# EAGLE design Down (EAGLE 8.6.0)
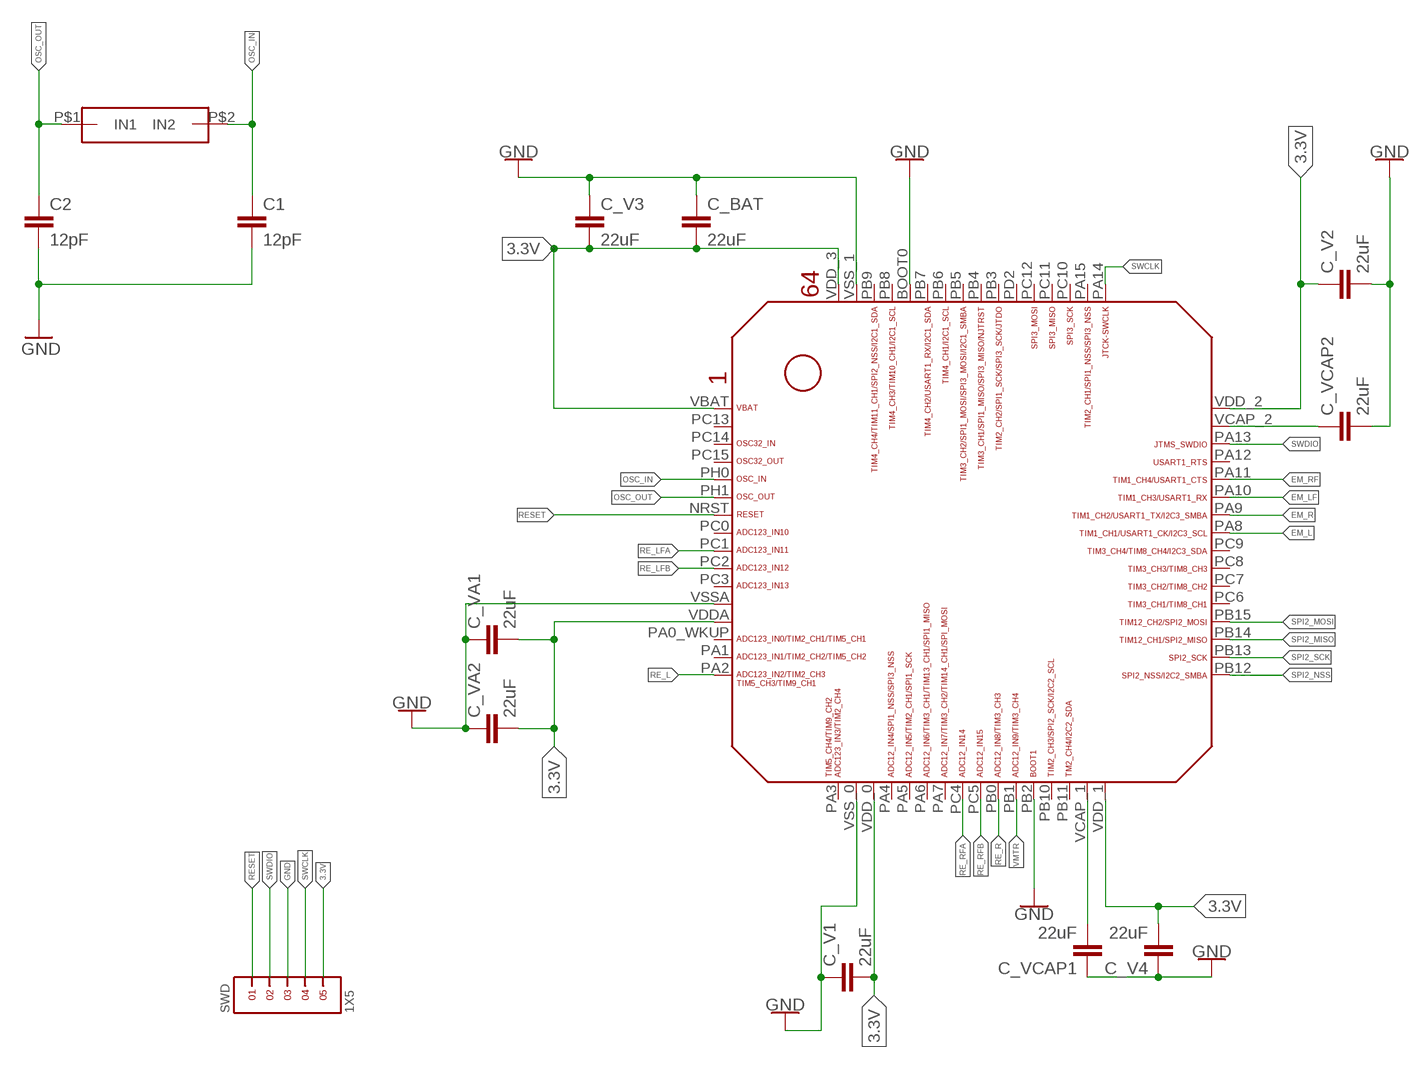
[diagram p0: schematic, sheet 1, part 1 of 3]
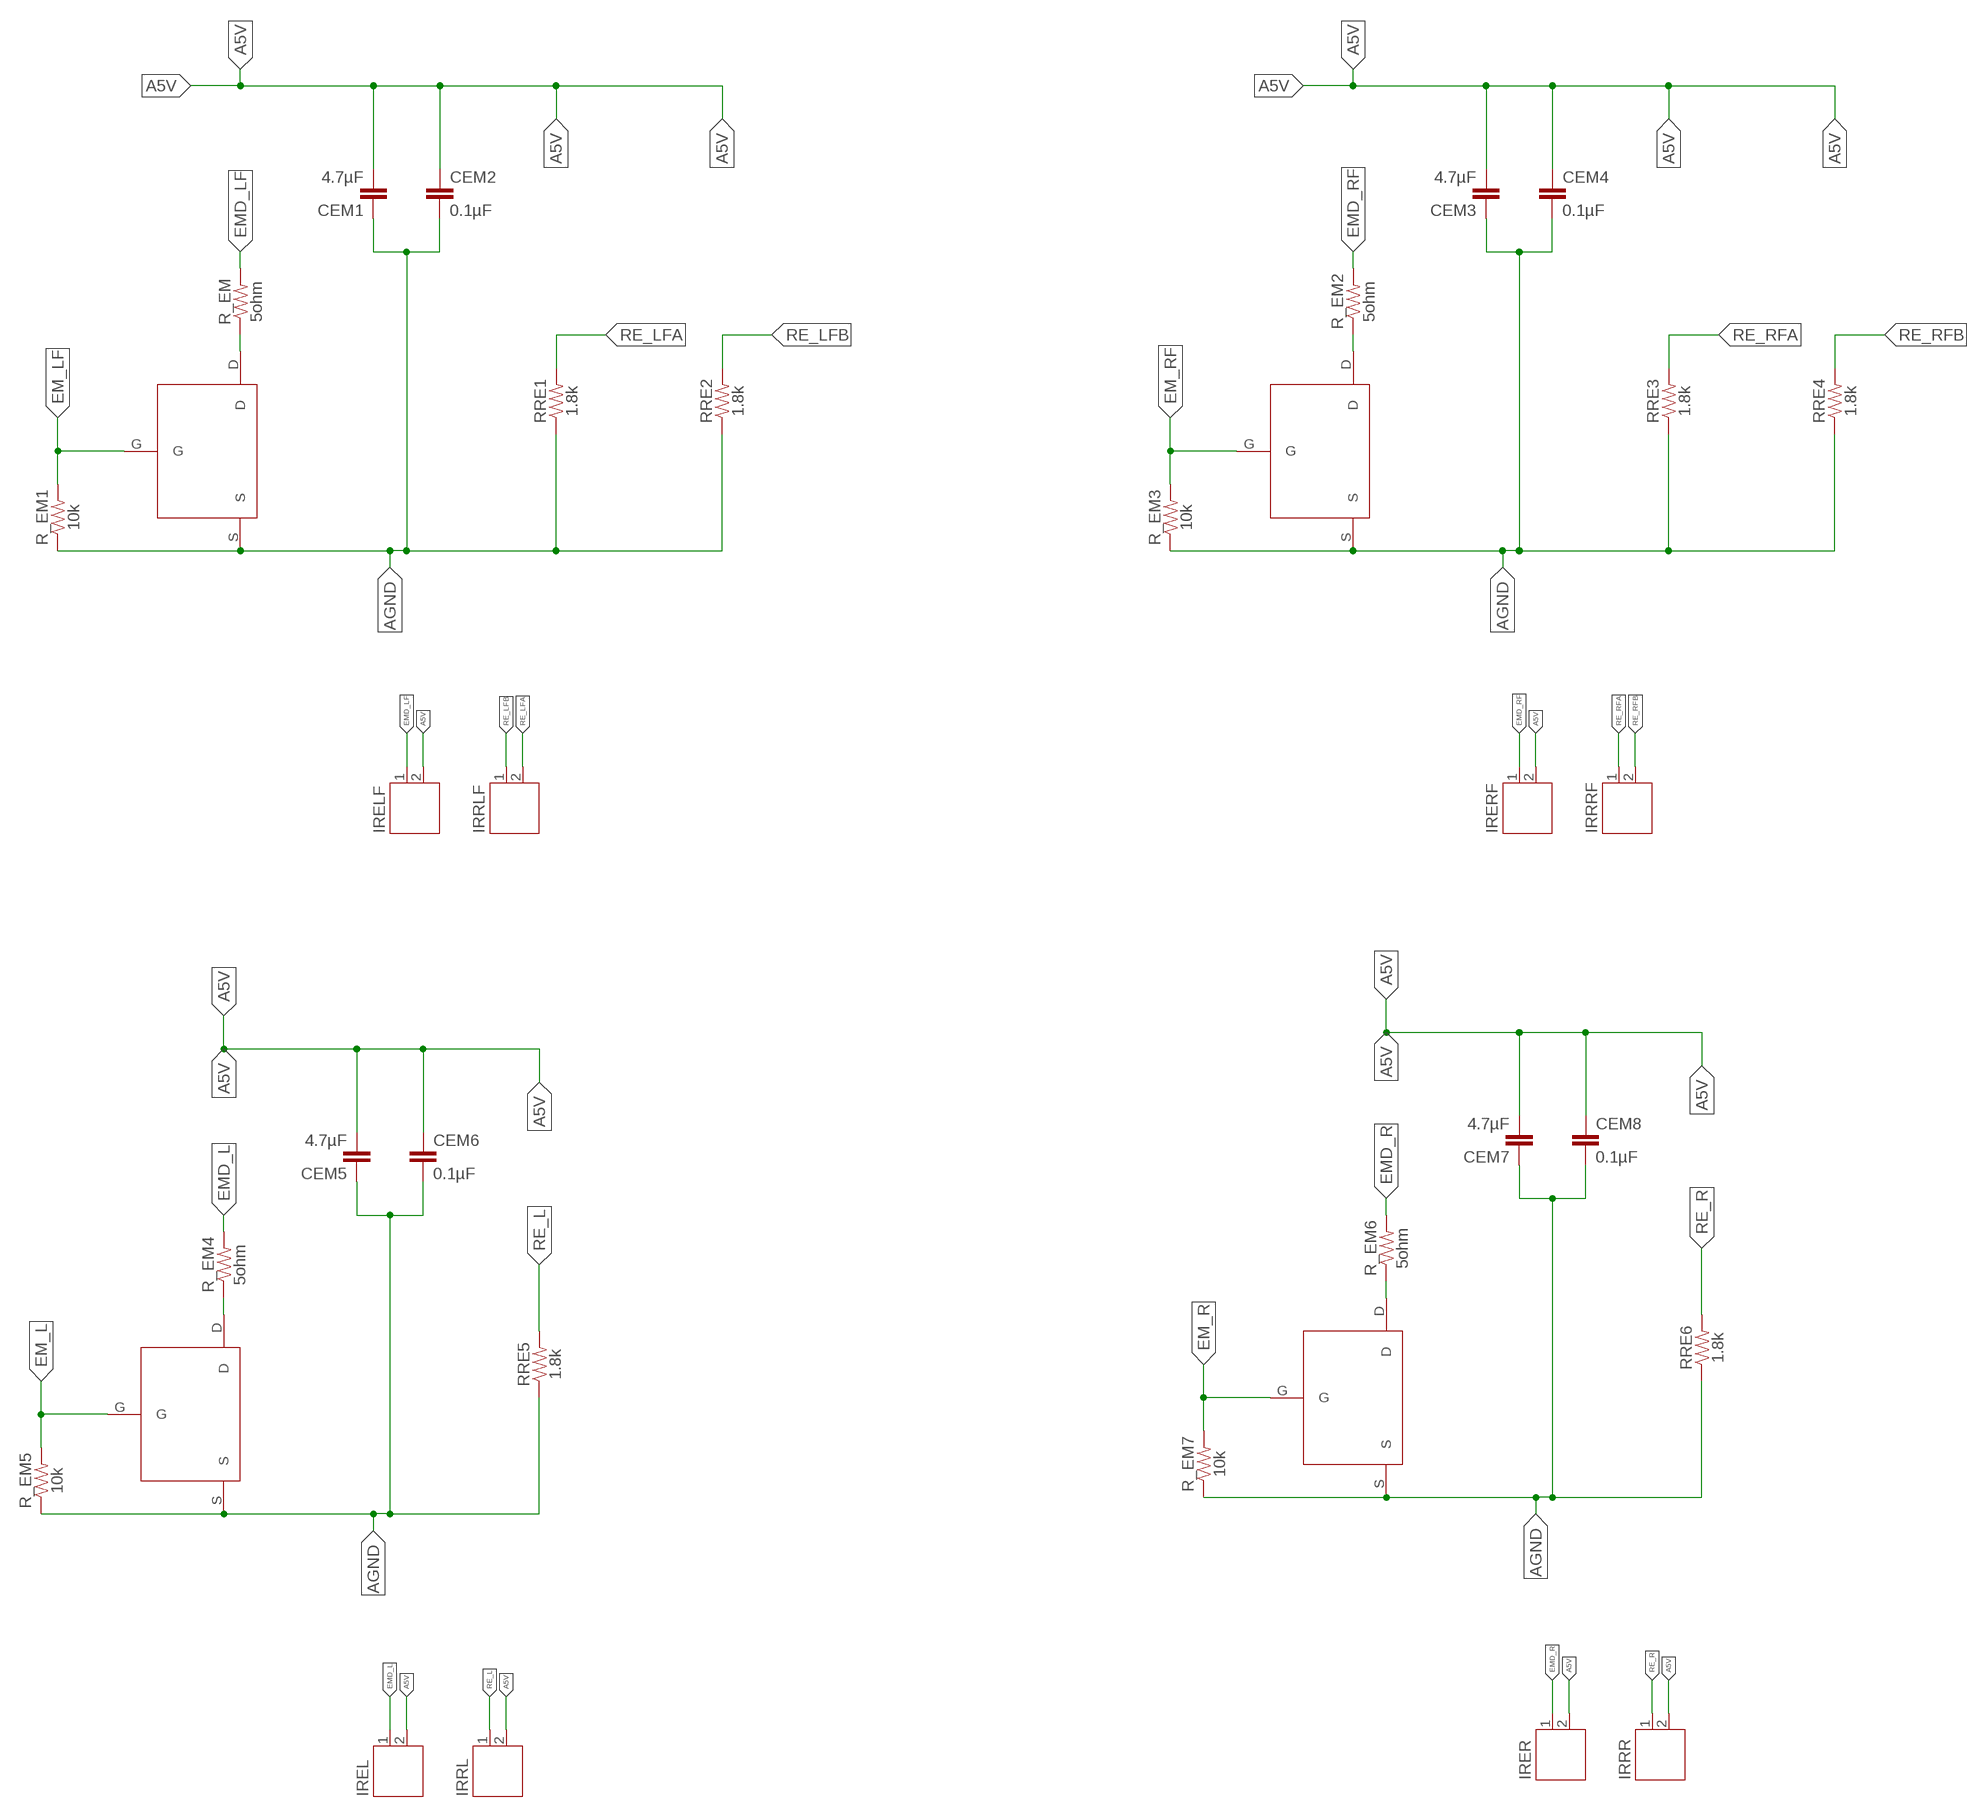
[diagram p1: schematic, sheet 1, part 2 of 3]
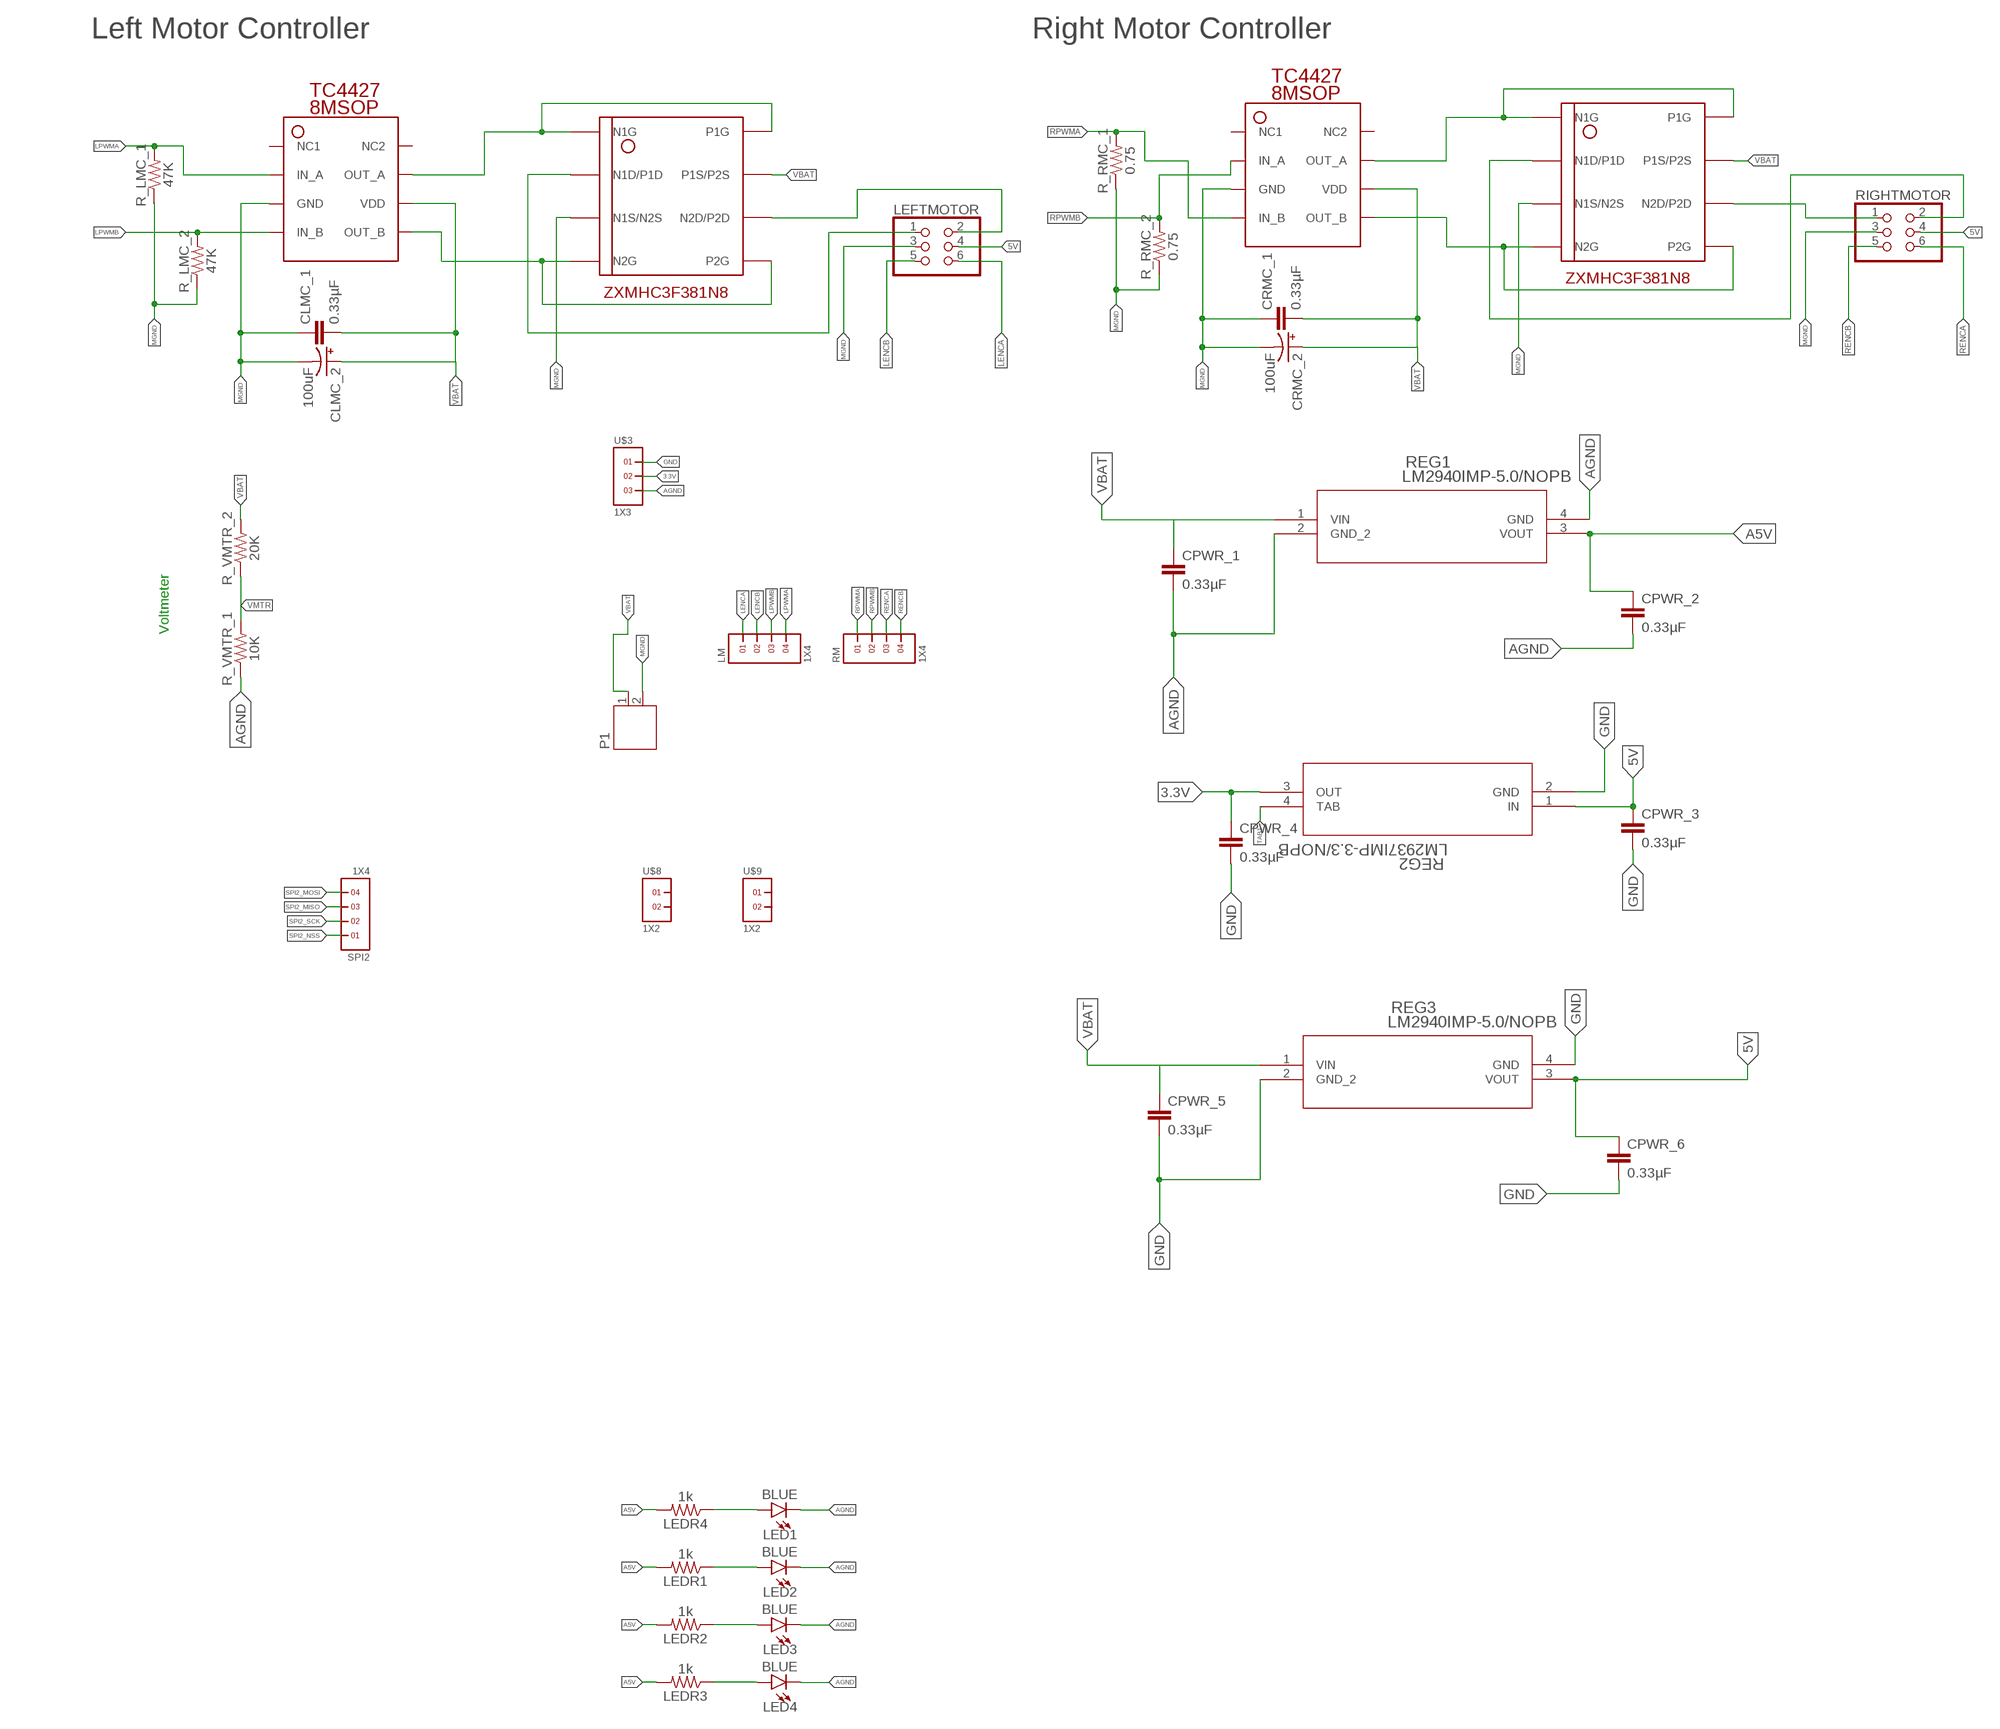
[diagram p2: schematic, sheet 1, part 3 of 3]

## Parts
C1  12pF  22PF-0603-50V-5%  [0603]
C2  12pF  22PF-0603-50V-5%  [0603]
C_BAT  22uF  22UF-0805-6.3V-20%  [0805]
C_V1  22uF  22UF-0805-6.3V-20%  [0805]
C_V2  22uF  22UF-0805-6.3V-20%  [0805]
C_V3  22uF  22UF-0805-6.3V-20%  [0805]
C_V4  22uF  22UF-0805-6.3V-20%  [0805]
C_VA1  22uF  22UF-0805-6.3V-20%  [0805]
C_VA2  22uF  22UF-0805-6.3V-20%  [0805]
C_VCAP1  22uF  22UF-0805-6.3V-20%  [0805]
C_VCAP2  22uF  22UF-0805-6.3V-20%  [0805]
CEM1  4.7µF  0.33UF/330NF-0805-50V-10%  [0805]
CEM2  0.1µF  0.33UF/330NF-0805-50V-10%  [0805]
CEM3  4.7µF  0.33UF/330NF-0805-50V-10%  [0805]
CEM4  0.1µF  0.33UF/330NF-0805-50V-10%  [0805]
CEM5  4.7µF  0.33UF/330NF-0805-50V-10%  [0805]
CEM6  0.1µF  0.33UF/330NF-0805-50V-10%  [0805]
CEM7  4.7µF  0.33UF/330NF-0805-50V-10%  [0805]
CEM8  0.1µF  0.33UF/330NF-0805-50V-10%  [0805]
CLMC_1  0.33µF  0.33UF/330NF-0805-50V-10%  [0805]
CLMC_2  100uF  100UF-POLAR-EIA7343-10V-10%(TANT)  [EIA7343]
CPWR_1  0.33µF  0.33UF/330NF-0805-50V-10%  [0805]
CPWR_2  0.33µF  0.33UF/330NF-0805-50V-10%  [0805]
CPWR_3  0.33µF  0.33UF/330NF-0805-50V-10%  [0805]
CPWR_4  0.33µF  0.33UF/330NF-0805-50V-10%  [0805]
CPWR_5  0.33µF  0.33UF/330NF-0805-50V-10%  [0805]
CPWR_6  0.33µF  0.33UF/330NF-0805-50V-10%  [0805]
CRMC_1  0.33µF  0.33UF/330NF-0805-50V-10%  [0805]
CRMC_2  100uF  100UF-POLAR-EIA7343-10V-10%(TANT)  [EIA7343]
IREL  JST-PH2  [JST-PH2]
IRELF  JST-PH2  [JST-PH2]
IRER  JST-PH2  [JST-PH2]
IRERF  JST-PH2  [JST-PH2]
IRRL  JST-PH2  [JST-PH2]
IRRLF  JST-PH2  [JST-PH2]
IRRR  JST-PH2  [JST-PH2]
IRRRF  JST-PH2  [JST-PH2]
LED1  BLUE  LED-BLUE1206  [LED-1206]
LED2  BLUE  LED-BLUE1206  [LED-1206]
LED3  BLUE  LED-BLUE1206  [LED-1206]
LED4  BLUE  LED-BLUE1206  [LED-1206]
LEDR1  1k  0.75OHM-0805-1/4W-1%  [0805]
LEDR2  1k  0.75OHM-0805-1/4W-1%  [0805]
LEDR3  1k  0.75OHM-0805-1/4W-1%  [0805]
LEDR4  1k  0.75OHM-0805-1/4W-1%  [0805]
LEFTMOTOR  PINHD-2X3  [2X03]
LM  1X4  [1X4]
P1  JST-PH2  [JST-PH2]
R_EM  5ohm  0.75OHM-0805-1/4W-1%  [0805]
R_EM1  10k  0.75OHM-0805-1/4W-1%  [0805]
R_EM2  5ohm  0.75OHM-0805-1/4W-1%  [0805]
R_EM3  10k  0.75OHM-0805-1/4W-1%  [0805]
R_EM4  5ohm  0.75OHM-0805-1/4W-1%  [0805]
R_EM5  10k  0.75OHM-0805-1/4W-1%  [0805]
R_EM6  5ohm  0.75OHM-0805-1/4W-1%  [0805]
R_EM7  10k  0.75OHM-0805-1/4W-1%  [0805]
R_LMC_1  47K  0.75OHM-0805-1/4W-1%  [0805]
R_LMC_2  47K  0.75OHM-0805-1/4W-1%  [0805]
R_RMC_1  0.75  0.75OHM-0805-1/4W-1%  [0805]
R_RMC_2  0.75  0.75OHM-0805-1/4W-1%  [0805]
R_VMTR_1  10K  0.75OHM-0805-1/4W-1%  [0805]
R_VMTR_2  20K  0.75OHM-0805-1/4W-1%  [0805]
REG1  LM2940IMP-5.0/NOPB  [MP04A]
REG2  LM2937IMP-3.3/NOPB  [MP04A]
REG3  LM2940IMP-5.0/NOPB  [MP04A]
RIGHTMOTOR  PINHD-2X3  [2X03]
RM  1X4  [1X4]
RRE1  1.8k  0.75OHM-0805-1/4W-1%  [0805]
RRE2  1.8k  0.75OHM-0805-1/4W-1%  [0805]
RRE3  1.8k  0.75OHM-0805-1/4W-1%  [0805]
RRE4  1.8k  0.75OHM-0805-1/4W-1%  [0805]
RRE5  1.8k  0.75OHM-0805-1/4W-1%  [0805]
RRE6  1.8k  0.75OHM-0805-1/4W-1%  [0805]
SPI2  1X4  [1X4]
SWD  1X5  [1X5]
U$1  STM32F405/415_LQFP64  [STM32F405/415_LQFP64]
U$2  OSC  [OSC]
U$3  1X3  [1X3]
U$4  MCH3474  [MCH3474]
U$5  MCH3474  [MCH3474]
U$6  MCH3474  [MCH3474]
U$7  MCH3474  [MCH3474]
U$8  1X2  [1X2]
U$9  1X2  [1X2]
U$15  TC4427(8MSOP)  [TC4427(8MSOP)]
U$16  ZXMHC3F381N8  [ZXMHC3F381N8]
U$17  TC4427(8MSOP)  [TC4427(8MSOP)]
U$18  ZXMHC3F381N8  [ZXMHC3F381N8]

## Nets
3.3V: C_BAT.2 C_V1.2 C_V2.1 C_V3.2 C_V4.2 C_VA1.2 C_VA2.2 CPWR_4.1 REG2.3(OUT) SWD.5 U$1.VBAT U$1.VDD_0 U$1.VDD_1 U$1.VDD_2 U$1.VDD_3 U$1.VDDA U$3.2
5V: CPWR_3.1 CPWR_6.1 LEFTMOTOR.4 REG2.1(IN) REG3.3(VOUT) RIGHTMOTOR.4
A5V: CEM1.2 CEM2.1 CEM3.2 CEM4.1 CEM5.2 CEM6.1 CEM7.2 CEM8.1 CPWR_2.1 IREL.2 IRELF.2 IRER.2 IRERF.2 IRRL.2 IRRR.2 LEDR1.2 LEDR2.2 LEDR3.2 LEDR4.2 REG1.3(VOUT)
AGND: CEM1.1 CEM2.2 CEM3.1 CEM4.2 CEM5.1 CEM6.2 CEM7.1 CEM8.2 CPWR_1.2 CPWR_2.2 LED1.C LED2.C LED3.C LED4.C R_EM1.1 R_EM3.1 R_EM5.1 R_EM7.1 R_VMTR_1.1 REG1.2(GND_2) REG1.4(GND) RRE1.1 RRE2.1 RRE3.1 RRE4.1 RRE5.1 RRE6.1 U$3.3 U$4.S U$5.S U$6.S U$7.S
EM_L: R_EM5.2 U$1.PA8 U$4.G
EM_LF: R_EM1.2 U$1.PA10 U$5.G
EM_R: R_EM7.2 U$1.PA9 U$7.G
EM_RF: R_EM3.2 U$1.PA11 U$6.G
EMD_L: IREL.1 R_EM4.2
EMD_LF: IRELF.1 R_EM.2
EMD_R: IRER.1 R_EM6.2
EMD_RF: IRERF.1 R_EM2.2
GND: C1.2 C2.2 C_BAT.1 C_V1.1 C_V2.2 C_V3.1 C_V4.1 C_VA1.1 C_VA2.1 C_VCAP1.1 C_VCAP2.2 CPWR_3.2 CPWR_4.2 CPWR_5.2 CPWR_6.2 REG2.2(GND) REG3.2(GND_2) REG3.4(GND) SWD.3 U$1.BOOT0 U$1.PB2 U$1.VSS_0 U$1.VSS_1 U$1.VSSA U$3.1
L: LEFTMOTOR.1 U$16.N1D/P1D
LENCA: LEFTMOTOR.6 LM.1
LENCB: LEFTMOTOR.5 LM.2
LPWMA: LM.4 R_LMC_1.2 U$15.IN_A
LPWMB: LM.3 R_LMC_2.2 U$15.IN_B
MGND: CLMC_1.1 CLMC_2.C(-) CRMC_1.1 CRMC_2.C(-) LEFTMOTOR.3 P1.2 R_LMC_1.1 R_LMC_2.1 R_RMC_1.1 R_RMC_2.1 RIGHTMOTOR.3 U$15.GND U$16.N1S/N2S U$17.GND U$18.N1S/N2S
N$1: R_EM.1 U$5.D
N$2: R_EM2.1 U$6.D
N$3: R_EM4.1 U$4.D
N$4: R_EM6.1 U$7.D
N$5: LED2.A LEDR1.1
N$6: LED3.A LEDR2.1
N$7: LED4.A LEDR3.1
N$8: LED1.A LEDR4.1
N$28: LEFTMOTOR.2 U$16.N2D/P2D
N$36: RIGHTMOTOR.1 U$18.N2D/P2D
OSC_IN: C1.1 U$1.PH0 U$2.P$2(IN2)
OSC_OUT: C2.1 U$1.PH1 U$2.P$1(IN1)
OUT_A: U$15.OUT_A U$16.N1G U$16.P1G
OUT_B: U$15.OUT_B U$16.N2G U$16.P2G
OUTA: U$17.OUT_A U$18.N1G U$18.P1G
OUTB: U$17.OUT_B U$18.N2G U$18.P2G
R: RIGHTMOTOR.2 U$18.N1D/P1D
RE_L: IRRL.1 RRE5.2 U$1.PA2
RE_LFA: IRRLF.2 RRE1.2 U$1.PC1
RE_LFB: IRRLF.1 RRE2.2 U$1.PC2
RE_R: IRRR.1 RRE6.2 U$1.PB0
RE_RFA: IRRRF.1 RRE3.2 U$1.PC4
RE_RFB: IRRRF.2 RRE4.2 U$1.PC5
RENCA: RIGHTMOTOR.6 RM.3
RENCB: RIGHTMOTOR.5 RM.4
RESET: SWD.1 U$1.NRST
RPWMA: R_RMC_1.2 RM.1 U$17.IN_B
RPWMB: R_RMC_2.2 RM.2 U$17.IN_A
SPI2_MISO: SPI2.3 U$1.PB14
SPI2_MOSI: SPI2.4 U$1.PB15
SPI2_NSS: SPI2.1 U$1.PB12
SPI2_SCK: SPI2.2 U$1.PB13
SWCLK: SWD.4 U$1.PA14
SWDIO: SWD.2 U$1.PA13
TAB1: REG2.4(TAB)
VBAT: CLMC_1.2 CLMC_2.A(+) CPWR_1.1 CPWR_5.1 CRMC_1.2 CRMC_2.A(+) P1.1 R_VMTR_2.2 REG1.1(VIN) REG3.1(VIN) U$15.VDD U$16.P1S/P2S U$17.VDD U$18.P1S/P2S
VCAP_1: C_VCAP1.2 U$1.VCAP_1
VCAP_2: C_VCAP2.1 U$1.VCAP_2
VMTR: R_VMTR_1.2 R_VMTR_2.1 U$1.PB1
Unconnected: U$1.PA0_WKUP(PA0_AKUP) U$1.PA1 U$1.PA3 U$1.PA4 U$1.PA5 U$1.PA6 U$1.PA7 U$1.PA12 U$1.PA15 U$1.PB3 U$1.PB4 U$1.PB5 U$1.PB6 U$1.PB7 U$1.PB8 U$1.PB9 U$1.PB10 U$1.PB11 U$1.PC0 U$1.PC3 U$1.PC6 U$1.PC7 U$1.PC8 U$1.PC9 U$1.PC10 U$1.PC11 U$1.PC12 U$1.PC13 U$1.PC14 U$1.PC15 U$1.PD2 U$8.1 U$8.2 U$9.1 U$9.2 U$15.NC1 U$15.NC2 U$17.NC1 U$17.NC2

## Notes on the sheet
- Left Motor Controller | Right Motor Controller
- Voltmeter

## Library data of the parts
C1 C2 = SparkFun-Capacitors:22PF: 22pF ceramic capacitors; PROD_ID: CAP-07876; VALUE: 22pF
C_BAT C_V1-C_V4 C_VA1 C_VA2 C_VCAP1 C_VCAP2 = SparkFun-Capacitors:22UF: 22µF ceramic capacitors; PROD_ID: CAP-08402
CEM1-CEM8 = SparkFun-Capacitors:0.33UF/330NF: 0.33µF/330nF ceramic capacitors; PROD_ID: CAP-08469; VALUE: 0.33µF
CLMC_1 CPWR_1-CPWR_6 CRMC_1 = SparkFun-Capacitors:0.33UF/330NF: 0.33µF/330nF ceramic capacitors; PROD_ID: CAP-08469
CLMC_2 CRMC_2 = SparkFun-Capacitors:100UF-POLAR: 100µF polarized capacitors; PROD_ID: CAP-07890
IREL IRELF IRER IRERF IRRL IRRLF IRRR IRRRF P1 = jst-ph:JST-PH2
LED1-LED4 = SparkFun-LED:LED-BLUE: Blue SMD LED; PROD_ID: DIO-09911
LEDR1-LEDR4 R_EM R_EM1-R_EM7 R_LMC_1 R_LMC_2 R_VMTR_1 R_VMTR_2 RRE1-RRE6 = SparkFun-Resistors:0.75OHM: 0.75Ω resistor; PROD_ID: RES-08474; VALUE: 0.75
LEFTMOTOR RIGHTMOTOR = pinhead:PINHD-2X3: PIN HEADER
LM RM SPI2 = headers(2mm):1X4
R_RMC_1 R_RMC_2 = SparkFun-Resistors:0.75OHM: 0.75Ω resistor; PROD_ID: RES-08474
REG1 REG3 = LM2940IMP-5.0:LM2940IMP-5.0/NOPB; 3D_LIBRARY_NAME: National_LDO; BASE_PN: LM2940; COMP: TypeLDO; COPYRIGHT: Copyright C 2015 Accelerated Designs. All rights reserved; LIBRARY: ReferenceLM2940IMP; MANUFACTURER_PART_NUMBER: LM2940IMP5.0NOPB; PIN: Count4; SYMBOL: NameLM2940IMP50; TYPE: LM2940IMP5.0; VENDOR: National Semiconductor; VERSION: 1
REG2 = LM2937IMP-3.3:LM2937IMP-3.3/NOPB; COPYRIGHT: Copyright C 2015 Accelerated Designs. All rights reserved; MANUFACTURER_PART_NUMBER: lm2937imp3_3nopb; VENDOR: National Semiconductor
SWD = headers(2mm):1X5
U$1 = STM32F405RG:STM32F405/415_LQFP64
U$2 = Cristal Oscillator:OSC
U$3 = headers(2mm):1X3
U$4-U$7 = MCH3474:MCH3474
U$8 U$9 = headers(2mm):1X2
U$15 U$17 = TC4427(8MSOP):TC4427(8MSOP)
U$16 U$18 = ZXMHC3F381N8:ZXMHC3F381N8

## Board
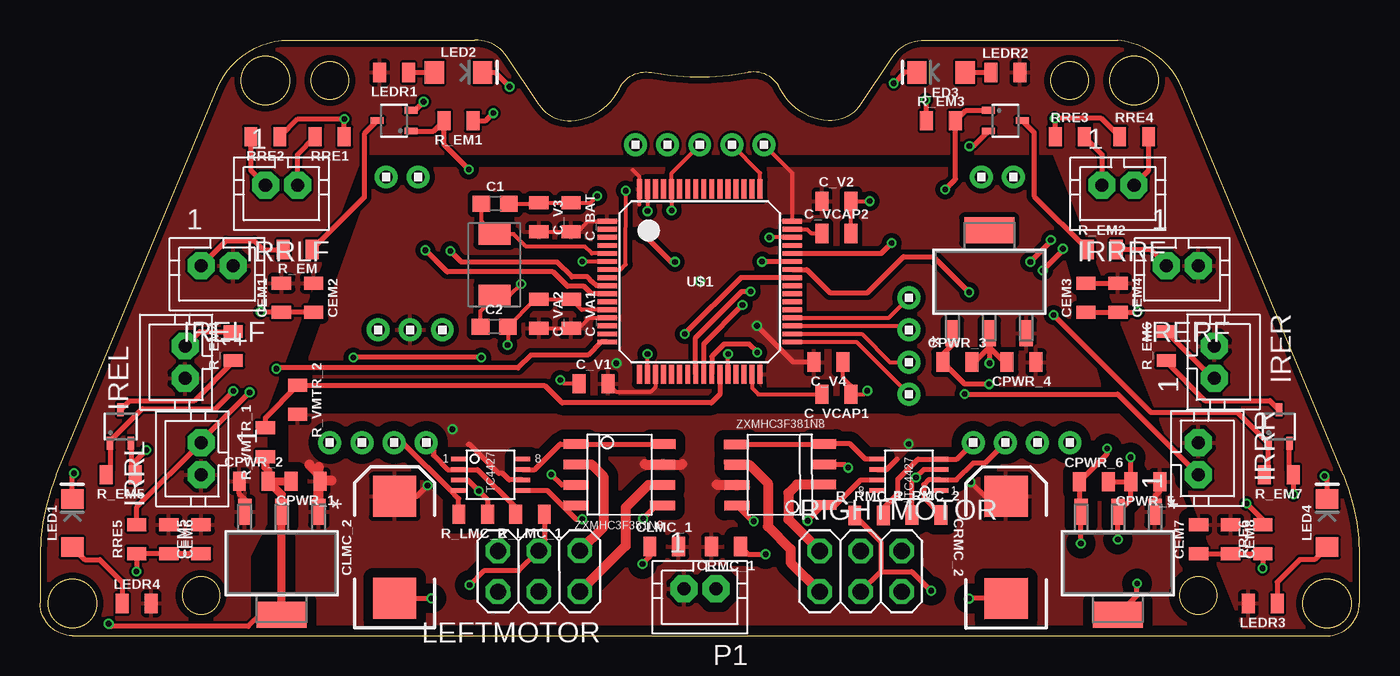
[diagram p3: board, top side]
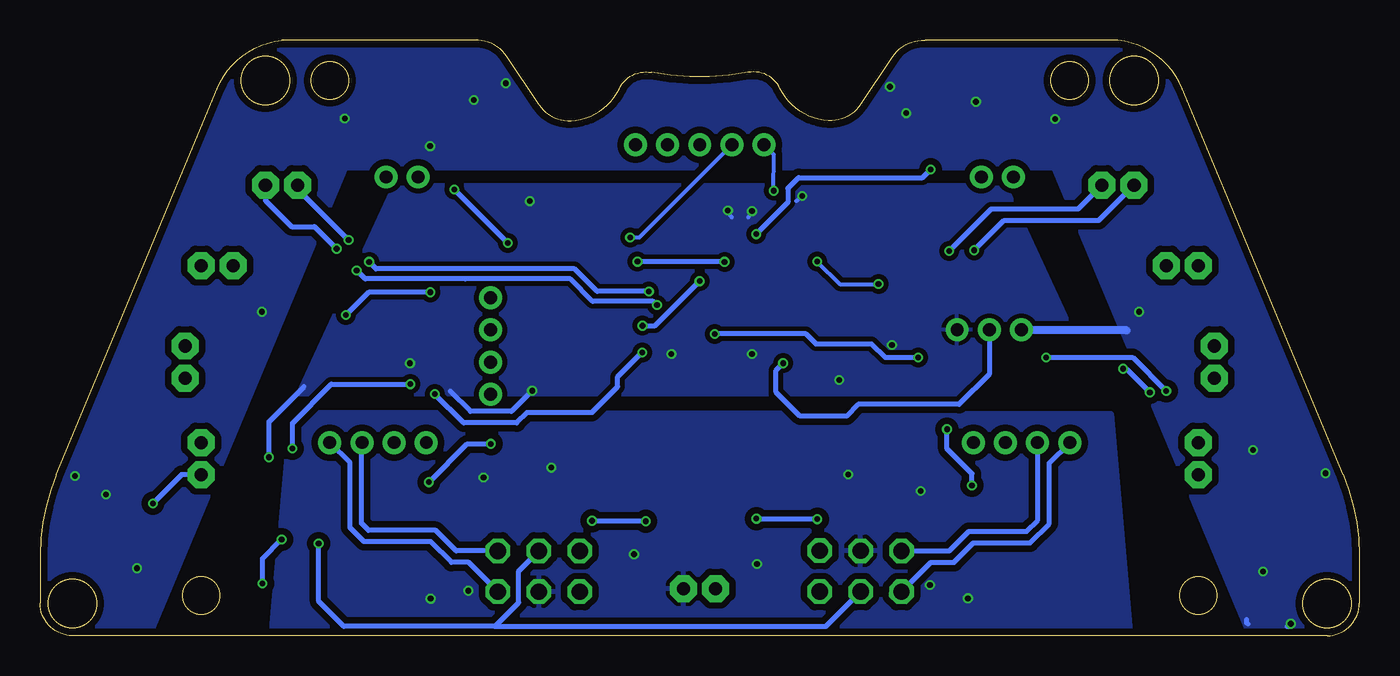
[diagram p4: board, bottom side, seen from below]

Size 82 x 37 mm. Coordinates in mm from the lower left corner, seen from the top.
Outline: 2,0 80,0 arc90 82,2 82,5 arc23 81,10 71,34 arc61 67,37 55,37 arc59 53,36 51,33 arc-59 49,32 arc-61 46,34 arc75 44,35 arc-22 38,35 arc75 36,34 arc-61 33,32 arc-59 31,33 29,36 arc59 27,37 15,37 arc61 11,34 1,10 arc23 0,5 0,2 arc90 2,0
Outline: circle at 10,2.5 radius 1.15
Outline: circle at 72,2.5 radius 1.15
Outline: circle at 14,34.5 radius 1.5
Outline: circle at 2,2 radius 1.5
Outline: circle at 80,2 radius 1.5
Outline: circle at 68,34.5 radius 1.5
Outline: circle at 18,34.5 radius 1.15
Outline: circle at 64,34.5 radius 1.15
Copper layers (1*16): Top 0.035559375mm / dielectric 1.6mm / Bottom 0.035559375mm
Design rules "oshpark-2layer *": minimum track width 6mil, minimum drill 10mil, track to track 6mil, track to pad 6mil, pad to pad 6mil, via to via 6mil, smd to smd 6mil, copper to edge 15mil, drill to drill 6mil, minimum pad ring 5mil, minimum via ring 5mil, stop-mask expansion 2.5mil, vias tented up to drill 12mil, thermal gap 10mil

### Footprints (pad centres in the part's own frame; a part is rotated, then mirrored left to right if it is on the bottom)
0603 = smd 1.1 x 1: 1 -0.85,0; 2 0.85,0
0805 = smd 0.8 x 1.2: 1 -0.9,0; 2 0.9,0
EIA7343 = smd 2.55 x 2.7: A 3.17,0; C -3.17,0
JST-PH2 = drill 0.813 pad 1.676 octagon: 1 1,0; 2 -1,0
LED-1206 = smd 1.2 x 1.4: A -1.5,0; C 1.5,0
2X03 = drill 1.016 octagon: 1 -2.54,-1.27; 2 -2.54,1.27; 3 0,-1.27; 4 0,1.27; 5 2.54,-1.27; 6 2.54,1.27
1X4 = drill 0.8 pad 1.422: 1 -3,0; 2 -1,0; 3 1,0; 4 3,0
MP04A = smd 1.6 x 0.838: 1 -3.2,2.3; 2 -3.2,0; 3 -3.2,-2.3 | smd 1.6 x 3.099: 4 3.2,0
1X5 = drill 0.8 pad 1.422: 1 -4,0; 2 -2,0; 3 0,0; 4 2,0; 5 4,0
STM32F405/415_LQFP64 = smd 0.3 x 1.2: BOOT0 -1.75,5.75; PA3 -3.75,-5.75; PA4 -2.25,-5.75; PA5 -1.75,-5.75; PA6 -1.25,-5.75; PA7 -0.75,-5.75; PA14 3.75,5.75; PA15 3.25,5.75; PB0 0.75,-5.75; PB1 1.25,-5.75; PB2 1.75,-5.75; PB3 0.75,5.75; PB4 0.25,5.75; PB5 -0.25,5.75; PB6 -0.75,5.75; PB7 -1.25,5.75; PB8 -2.25,5.75; PB9 -2.75,5.75; PB10 2.25,-5.75; PB11 2.75,-5.75; PC4 -0.25,-5.75; PC5 0.25,-5.75; PC10 2.75,5.75; PC11 2.25,5.75; PC12 1.75,5.75; PD2 1.25,5.75; VCAP_1 3.25,-5.75; VDD_0 -2.75,-5.75; VDD_1 3.75,-5.75; VDD_3 -3.75,5.75; VSS_0 -3.25,-5.75; VSS_1 -3.25,5.75 | smd 1.2 x 0.3: NRST -5.75,0.75; PA0_WKUP -5.75,-2.75; PA1 -5.75,-3.25; PA2 -5.75,-3.75; PA8 5.75,0.25; PA9 5.75,0.75; PA10 5.75,1.25; PA11 5.75,1.75; PA12 5.75,2.25; PA13 5.75,2.75; PB12 5.75,-3.75; PB13 5.75,-3.25; PB14 5.75,-2.75; PB15 5.75,-2.25; PC0 -5.75,0.25; PC1 -5.75,-0.25; PC2 -5.75,-0.75; PC3 -5.75,-1.25; PC6 5.75,-1.75; PC7 5.75,-1.25; PC8 5.75,-0.75; PC9 5.75,-0.25; PC13 -5.75,3.25; PC14 -5.75,2.75; PC15 -5.75,2.25; PH0 -5.75,1.75; PH1 -5.75,1.25; VBAT -5.75,3.75; VCAP_2 5.75,3.25; VDD_2 5.75,3.75; VDDA -5.75,-2.25; VSSA -5.75,-1.75
OSC = smd 1.3 x 2: P$1 0,0.1; P$2 3.8,0.1
1X3 = drill 0.8 pad 1.422: 1 -2,0; 2 0,0; 3 2,0
MCH3474 = smd 0.406 x 0.813: D 0,1.05; G -0.65,-1.05; S 0.65,-1.05
1X2 = drill 0.8 pad 1.422: 1 -1,0; 2 1,0
TC4427(8MSOP) = smd 0.95 x 0.3: GND -1.975,-0.325; IN_A -1.975,0.325; IN_B -1.975,-0.975; NC1 -1.975,0.975; NC2 1.975,0.975; OUT_A 1.975,0.325; OUT_B 1.975,-0.975; VDD 1.975,-0.325
ZXMHC3F381N8 = smd 0.6 x 1.55: N1D/P1D -0.635,-2.7; N1G -1.905,-2.7; N1S/N2S 0.635,-2.7; N2D/P2D 0.635,2.7; N2G 1.905,-2.7; P1G -1.905,2.7; P1S/P2S -0.635,2.7; P2G 1.905,2.7

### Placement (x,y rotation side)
C1  28.28,26.84 0 top
C2  28.22,19.2 0 top
C_BAT  33,26 270 top
C_V1  34.4,15.66 0 top
C_V2  49.5,27 0 top
C_V3  31,26 270 top
C_V4  49,17 180 top
C_VA1  33.01,20 270 top
C_VA2  31,20 270 top
C_VCAP1  49.5,15 180 top
C_VCAP2  49.5,25 0 top
CEM1  15,21 90 top
CEM2  17,21 270 top
CEM3  65,21 90 top
CEM4  67,21 270 top
CEM5  10,6 90 top
CEM6  8,6 270 top
CEM7  72,5.99 90 top
CEM8  74,6 270 top
CLMC_1  38.79,5.54 0 top
CLMC_2  22.03,5.49 90 top
CPWR_1  16.5,9.6 180 top
CPWR_2  13.28,9.6 0 top
CPWR_3  57.01,17 0 top
CPWR_4  61,17 180 top
CPWR_5  68.69,9.56 180 top
CPWR_6  65.5,9.56 0 top
CRMC_1  42.63,5.54 180 top
CRMC_2  60.05,5.48 90.1 top
IREL  9,17 90 top
IRELF  11,23 180 top
IRER  73,17 270 top
IRERF  71,23 180 top
IRRL  10,11 90 top
IRRLF  15,28 180 top
IRRR  72,11 270 top
IRRRF  67,28 180 top
LED1  2,7 90 top
LED2  26,35 0 top
LED3  56,35 180 top
LED4  80,7 90 top
LEDR1  22,35 180 top
LEDR2  60,35 0 top
LEDR3  76,2 180 top
LEDR4  6,2 0 top
LEFTMOTOR  31,4 180.1 top
LM  21,12 0 top
P1  41.01,2.92 180 top
R_EM  16,24 180 top
R_EM1  26,32 180 top
R_EM2  66,24 0 top
R_EM3  56,32 0 top
R_EM4  12,18 90 top
R_EM5  5,10 180 top
R_EM6  70,18 90 top
R_EM7  77,10 180 top
R_LMC_1  30.44,7.55 180 top
R_LMC_2  26.92,7.54 180 top
R_RMC_1  51.53,7.47 0 top
R_RMC_2  55.1,7.49 0 top
R_VMTR_1  14,12.01 90 top
R_VMTR_2  16,14.65 270 top
REG1  15.01,4.5 270 top
REG2  59,22 90 top
REG3  67,4.5 270 top
RIGHTMOTOR  51,4 0 top
RM  61,12 0 top
RRE1  18,31 180 top
RRE2  14,31 180 top
RRE3  64,31 0 top
RRE4  68,31 0 top
RRE5  6,6 90 top
RRE6  76,6 90 top
SPI2  54,18 90 top
SWD  41,30.5 0 top
U$1  41,22 0 top
U$2  28.34,21.15 90 top
U$3  23,19 180 top
U$4  5,13 0 top
U$5  22,32 90 top
U$6  60,32 270 top
U$7  77,13 0 top
U$8  22.5,28.5 0 top
U$9  59.5,28.5 0 top
U$15  28,10 0 top
U$16  36,10 269.9 top
U$17  54,10 180 top
U$18  46,10 90.3 top

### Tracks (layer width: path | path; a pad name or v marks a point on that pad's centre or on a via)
3.3V  (via drill 0.35)
  Top 0.254: C_V3.2 C_BAT.2 33.42,25.1 34.07,25.75 U$1.VBAT | C_VA2.2 C_VA1.2 33.49,19.1 34.14,19.75 U$1.VDDA | U$1.VDD_0 38.25,15.44 37.98,15.17 35.79,15.17 C_V1.2 | 37.24,26.78 U$1.VDD_3 37.25,28.53 36.85,28.93 | U$1.VDD_2 46.75,28.75 SWD.5
  Top 0.305: v44.56,19.26 45.84,17.98 45.84,17.97 46.82,17 C_V4.2
  Bottom 0.305: U$3.2 23,16.25 24.88,14.37 31.16,14.37 31.88,13.65 34.77,13.65 36.26,15.14 36.26,16.49 v35.82,16.93 | v44.56,19.26 43.78,19.26 v41.01,22.03
  pour Top (isolate 0.305): 16,15 21,29 62,29 66,15
5V  (via drill 0.35)
  Top 0.305: v64.69,5.73 REG3.3 64.6,7.8 CPWR_6.1 66.32,11.28 v66.32,11.63 | REG2.1 56.71,18.08 56.11,17.48 CPWR_3.1 57.48,15.63 v58.99,15.63
  Bottom 0.305: 53.74,0.57 63.13,0.57 64.69,2.13 v64.69,5.73 | 53.74,0.57 52.26,2.05 52.26,4.01 RIGHTMOTOR.4 | 53.74,0.57 33.16,0.57 LEFTMOTOR.4 | v66.32,11.63 66.32,13.21 63.9,15.63 v58.99,15.63
A5V
  Top 0.305: REG1.3 12.71,8.49 12.38,8.82 CPWR_2.1 | CEM3.2 CEM4.1
  pour Top: 13,-1 13,5 14,7 14,14 20,30 63,30 75,0 76,-2 91,-2 72,42 10,42 -10,-1
AGND  (via drill 0.35)
  Top 0.305: CPWR_2.2 14.42,9.6 | REG1.4 13.66,1.3 12.93,0.57 4.43,0.57 v4.26,0.74 | RRE1.1 v18.9,32.11 16.01,32.11 RRE2.1 | U$5.S 23.3,32.65 v23.83,33.18 | R_EM1.1 27.69,32 v28.16,32.47 | CEM2.2 CEM1.1 13.72,20.1 v13.69,20.13 | CEM3.1 CEM4.2 68.18,20.1 v68.21,20.13 | RRE3.1 63.1,32.11 v63.07,32.14 65.96,32.14 RRE4.1 | R_EM3.1 55.1,33.24 v55.05,33.29 | U$6.S 58.02,30.42 v57.76,30.42 | U$4.S 5.65,10.25 R_EM5.1 5.9,10.83 v6.6,11.53 | CEM5.1 CEM6.2 RRE5.1 6,4 v5.98,3.98 | CEM7.1 CEM8.2 RRE6.1 v76,4.2 v75.99,4.19 | v77.91,8.78 v77.9,8.79 R_EM7.1 77.65,10.25 U$7.S | LED1.C 2,10 v2.09,10.09 | LED4.C 80,9.76 v79.84,9.92 | LED3.C 53.73,35 v53.06,34.33 | LED2.C 28.29,35 v29.18,34.11
  Top 0.508: CPWR_2.2 14.18,10.26 14,10.44 R_VMTR_1.1 | CPWR_2.2 CPWR_1.2 | CPWR_2.2 15.01,8.77 REG1.2 REG1.4
  Bottom 0.305: 6.93,0.72 7,0.79 7,1 | v4.26,0.74 4.43,0.57 4.5,0.57
  Bottom 0.508: U$3.3 14.52,19 14.47,18.95
  pour Bottom (isolate 0.406): 6,-2 19,29 63,29 76,-2 89,-2 70,44 11,44 -8,-2
EM_L  (via drill 0.35)
  Top 0.305: v27.43,17.29 v19.47,17.29 | v12,15.2 10.91,14.11 6.35,14.11 4.35,12.11 U$4.G 4.35,10.25 R_EM5.2 | v40.06,18.75 43.56,22.25 U$1.PA8
  Bottom 0.305: v40.06,18.75 34.39,18.75 33.78,18.14 30.32,18.14 29.47,17.29 v27.43,17.29 | v19.47,17.29 14.09,17.29 v12,15.2
EM_LF  (via drill 0.35)
  Top 0.305: U$5.G 24.45,31.35 R_EM1.2 25.1,30.51 v26.65,28.96 | U$1.PA10 v44.88,23.25 v44.87,23.24 | v37.49,24.95 39.21,23.23 v39.46,23.23
  Bottom 0.305: v26.65,28.96 27.15,28.46 34.86,28.46 35.52,27.8 35.52,26.92 v37.49,24.95 | v39.46,23.23 v44.86,23.23 v44.87,23.24
EM_R  (via drill 0.35)
  Top 0.305: R_EM7.2 76.35,10.25 U$7.G 74.43,13.87 69.05,13.87 v63,19.92 | U$1.PA9 47.65,22.75 49.08,21.32 51.43,21.32 53.67,23.56 55.52,23.56 v57.74,21.34
  Bottom 0.305: v57.74,21.34 61.58,21.34 v63,19.92
EM_RF  (via drill 0.35)
  Top 0.305: U$6.G 57.55,32.65 R_EM3.2 56.9,28.37 v56.26,27.73 | U$1.PA11 52.28,23.75 v52.93,24.4
  Bottom 0.305: v52.93,24.4 v56.26,27.73
EMD_L
  Top 0.305: IREL.1 9.9,18.9 R_EM4.2
EMD_LF
  Top 0.305: IRELF.1 11.55,24.55 13.3,24.55 13.87,23.98 15.08,23.98 R_EM.2
EMD_R
  Top 0.305: R_EM6.2 72.9,16 IRER.1
EMD_RF
  Top 0.305: R_EM2.2 69,24 IRERF.1
GND  (via drill 0.35)
  Top 0.254: C1.2 30.94,26.84 C_V3.1 C_BAT.1 34.21,26.9 v34.63,27.32 | C_V4.1 49.91,16.03 50.4,15.54 C_VCAP1.1 51.2,15 v51.42,15.22 | U$1.VSS_0 v37.75,17.51 | v29.05,18.06 29.07,18.08 C2.2 30.77,20.9 C_VA2.1 C_VA1.1 33.66,20.25 U$1.VSSA | C_V1.1 32.56,15.66 v32.33,15.89 | U$1.PB2 v42.75,17.5 v42.76,17.51 | SWD.3 39.25,28.75 U$1.BOOT0 v39.25,26.42 | U$1.VSS_1 v37.75,26.38 | C_VCAP2.2 C_V2.2 v51.57,27
  Top 0.305: CPWR_6.2 CPWR_5.2 | CPWR_5.2 67.79,8.49 REG3.2 v66.99,5.98 | CPWR_3.2 58.07,17 59,17.93 | 59,17.93 REG2.2 | CPWR_4.2 59.93,17 59,17.93 | 59,17.93 v59,16.94 v59.01,16.93 | CPWR_5.2 v67.79,11.08 v67.78,11.09 | REG3.4 68.18,2.48 v68.18,3.24
  Bottom 0.254: v34.63,27.32 34.68,27.32 35,27 | v39.25,26.42 39.25,26.25 39,26 | v37.75,26.38 37.75,26.25 38,26
  Bottom 0.305: v67.78,11.09 67.78,13.3 65.6,15.48 | v68.18,3.24 68.18,4.79 v66.99,5.98 | v51.42,15.22 52.7,13.94 55.25,13.94 56.51,15.2
  pour Bottom (isolate 0.305): 16,15 22,28 60,28 66,15
L
  Top 0.61: U$16.N1D/P1D 34.27,10.64 35.01,9.9 35.01,6.75 LEFTMOTOR.1
LENCA
  Bottom 0.305: LM.1 19.27,10.73 19.27,6.96 20.47,5.76 24,5.76 25.2,4.56 26.63,4.56 LEFTMOTOR.6
LENCB
  Bottom 0.305: LM.2 19.99,7.18 20.69,6.48 24.28,6.48 25.49,5.27 LEFTMOTOR.5
LPWMA
  Top 0.305: LM.4 24.44,11.56 24.44,11.2 25.31,10.32 U$15.IN_A 27.19,10.32 29.54,7.97 R_LMC_1.2
LPWMB
  Top 0.305: 22.39,12 LM.3 22.53,12 25.51,9.02 | 25.51,9.02 U$15.IN_B | R_LMC_2.2 26.02,8.51 25.51,9.02
MGND  (via drill 0.35)
  Top 0.305: CLMC_2.C v24.33,2.32 | U$15.GND 26.58,9.68 v27.26,8.99 27.83,8.42 27.82,8.41 R_LMC_2.1 | R_LMC_1.1 31.34,5.62 LEFTMOTOR.3 29.74,4.02 27.57,4.02 v26.69,3.14 | U$16.N1S/N2S 32.41,9.37 v31.77,10.01 | U$18.N1S/N2S 50.02,10.65 v50.23,10.44 | R_RMC_1.1 52.26,5.84 52.26,3.99 | 52.26,3.99 RIGHTMOTOR.3 | CRMC_2.C v57.74,2.31 v57.73,2.3 | U$17.GND 54.94,10.32 v54.44,9.83 54.2,9.59 R_RMC_2.1 | 52.26,3.99 54.18,3.99 v55.38,2.79 | v37.44,4.45 37.89,4.9 CLMC_1.1 | CRMC_1.1 44.01,5.06 v45.09,5.06
  pour Bottom (isolate 0.406): 15.42,13.81 14,-2.27 67.82,-2.03 66.4,13.9
N$1
  Top 0.305: U$5.D 20.14,31.19 20.14,27.24 R_EM.1
N$2
  Top 0.305: U$6.D 61.78,31.27 61.78,27.32 R_EM2.1
N$3
  Top 0.305: R_EM4.1 12,17.01 9.57,14.58 5.53,14.58 U$4.D
N$4
  Top 0.305: R_EM6.1 70,17.01 72.41,14.6 76.45,14.6 U$7.D
N$5
  Top 0.305: LEDR1.1 LED2.A
N$6
  Top 0.305: LED3.A LEDR2.1
N$7
  Top 0.305: LED4.A 79.22,4.72 78.29,4.72 76.9,3.34 LEDR3.1
N$8
  Top 0.305: LED1.A 2.78,4.72 3.71,4.72 5.1,3.34 LEDR4.1
N$28
  Top 0.61: U$16.N2D/P2D 37.79,9.36 36.39,7.96 36.39,5.59 LEFTMOTOR.2
N$36
  Top 0.61: U$18.N2D/P2D 44.09,10.62 45.23,9.48 45.23,6.79 46.65,5.37 46.65,4.54 RIGHTMOTOR.1
OSC_IN
  Top 0.254: U$1.PH0 34.29,23.75 33.86,24.18 30.21,24.18 29.44,24.95 U$2.P$2 27.43,25.76 C1.1
OSC_OUT  (via drill 0.35)
  Top 0.254: U$1.PH1 v33.7,23.25 | v29.89,21.85 29.19,21.15 28.35,21.15 | 28.35,21.15 U$2.P$1 | C2.1 27.37,20.17 28.35,21.15
  Bottom 0.254: v33.7,23.25 32.3,21.85 v29.89,21.85
OUT_A
  Top 0.305: U$15.OUT_A 30.74,10.32 32.32,11.9 U$16.N1G U$16.P1G
OUT_B  (via drill 0.35)
  Top 0.305: U$15.OUT_B 31.52,9.02 32.44,8.1 | 32.44,8.1 U$16.N2G | 32.44,8.1 33.3,7.24 v33.69,7.24 | v37.48,7.27 38.3,8.09 U$16.P2G
  Bottom 0.305: v33.69,7.24 37.45,7.24 v37.48,7.27
OUTA  (via drill 0.35)
  Top 0.305: U$18.N1G 49.44,8.11 51,9.68 U$17.OUT_A | 43.56,8.08 U$18.P1G 44.28,7.11 v44.35,7.11 | 48.49,8.11 U$18.N1G | v47.7,7.14 48.67,8.11 U$18.N1G
  Bottom 0.305: v44.35,7.11 47.67,7.11 v47.7,7.14
OUTB
  Top 0.305: U$18.P2G 48.66,11.89 U$18.N2G 50.34,11.92 51.28,10.98 U$17.OUT_B
R
  Top 0.61: U$18.N1D/P1D 47.03,9.38 46.5,8.85 46.5,7.23 RIGHTMOTOR.2
RE_L  (via drill 0.35)
  Top 0.305: U$1.PA2 34.86,18.25 34.04,17.43 30.51,17.43 29.72,16.64 14.74,16.64 v14.69,16.59 | v13.02,15.12 10,12.1 IRRL.1 6,8 RRE5.2
  Bottom 0.305: v14.69,16.59 14.49,16.59 v13.02,15.12
RE_LFA  (via drill 0.35)
  Top 0.305: U$1.PC1 34.57,21.75 34.34,21.97 34.34,21.98 34.03,22.29 33.05,22.29 32.13,23.21 26.19,23.21 v25.49,23.91 | IRRLF.2 16,29.9 RRE1.2
  Bottom 0.305: IRRLF.2 17.49,26.51 22.89,26.51 v25.49,23.91
RE_LFB  (via drill 0.35)
  Top 0.305: U$1.PC2 34.27,21.25 33.82,21.7 32.77,21.7 31.87,22.6 25.3,22.6 v23.95,23.95 | IRRLF.1 13.1,28.9 RRE2.2
  Bottom 0.305: v23.95,23.95 22.09,25.81 16.19,25.81 IRRLF.1
RE_R  (via drill 0.35)
  Top 0.305: v74.99,8.22 76,7.21 RRE6.2 | v57.47,15.01 66.99,15.01 IRRR.1 | U$1.PB0 41.75,17.36 42.51,18.12 44.07,18.12 44.07,18.11 v44.58,17.6
  Bottom 0.305: IRRR.1 73.21,10 v74.99,8.22 | v57.47,15.01 55.68,13.22 52.38,13.22 51.74,13.86 47.72,13.86 46.11,15.47 46.11,16.08 v44.59,17.6 v44.58,17.6
RE_RFA  (via drill 0.35)
  Top 0.305: RRE3.2 66,29.9 IRRRF.1 | v61.55,23.23 62.83,24.51 v62.83,24.58 | v44.16,21.39 43.62,21.39 40.75,18.52 U$1.PC4
  Bottom 0.305: v61.55,23.23 61.12,22.8 48.79,22.8 47.38,21.39 v44.16,21.39 | v62.83,24.58 66,27.75 IRRRF.1
RE_RFB  (via drill 0.35)
  Top 0.305: v62.33,22.7 63.57,23.94 v63.57,24.04 | RRE4.2 68.9,28.9 IRRRF.2 | U$1.PC5 41.25,18.14 v43.66,20.55
  Bottom 0.305: 55.56,22.17 55.57,22.18 | v62.33,22.7 61.8,22.17 55.56,22.17 | v63.57,24.04 64.95,25.42 66.38,25.42 68,27.04 IRRRF.2 | v43.66,20.55 43.89,20.78 47.65,20.78 49.04,22.17 55.56,22.17
RENCA
  Bottom 0.305: RIGHTMOTOR.6 56.14,5.27 57.42,6.55 61.6,6.55 62.02,6.97 62.02,11.98 RM.3
RENCB
  Bottom 0.305: RIGHTMOTOR.5 55.36,4.55 56.43,4.55 57.72,5.84 61.88,5.84 62.75,6.71 62.75,10.75 RM.4
RESET  (via drill 0.35)
  Top 0.254: U$1.NRST 36.08,22.75 36.4,23.07 v36.41,27.65
  Bottom 0.254: SWD.1 36.4,29.9 v36.41,27.65 36.41,27.85
RPWMA
  Top 0.305: R_RMC_1.2 52.43,7.93 53.31,8.81 53.31,9.72 54.56,10.98 U$17.IN_B 56.97,10.98 RM.1
RPWMB
  Top 0.305: R_RMC_2.2 54.92,8.57 54.92,9.38 55.22,9.68 U$17.IN_A 56.97,9.68 58.01,10.72 58.72,10.72 RM.2
SPI2_MISO
  Top 0.254: U$1.PB14 53.75,19.25 SPI2.3
SPI2_MOSI
  Top 0.254: U$1.PB15 52.75,19.75 SPI2.4
SPI2_NSS
  Top 0.254: U$1.PB12 50.75,18.25 SPI2.1
SPI2_SCK
  Top 0.254: U$1.PB13 51.07,18.75 52.83,16.99 SPI2.2
SWCLK
  Top 0.254: U$1.PA14 44.75,28.75 SWD.4
SWDIO  (via drill 0.35)
  Top 0.254: U$1.PA13 v45.33,24.75
  Bottom 0.254: v45.33,24.75 44.75,24.75 SWD.2
VBAT  (via drill 0.35)
  Top 0.305: 26.61,11.89 26.69,11.89 28.5,10.08 28.74,10.08 29.15,9.68 U$15.VDD | U$17.VDD 52.61,10.32 53.28,10.99 | CPWR_5.1 69.59,8.96 69.31,8.68 REG3.1 | CRMC_2.A 58.73,8.65 v57.84,9.54 | CLMC_2.A 23.4,8.66 v24.08,9.34
  Top 0.61: 37.57,10.66 37.6,10.63 U$16.P1S/P2S 39.88,10.63 39.92,10.67 | U$18.P1S/P2S 42.1,9.35 42.07,9.38 | REG1.1 17.31,10.46 17.33,10.48 | 18.09,9.65 17.45,9.65 CPWR_1.1 17.4,9.95 16.72,10.63
  Bottom 0.305: v24.08,9.34 24.08,10.07 25.62,11.61 v25.62,12.82 v25.63,12.83 | v53.98,11.92 55.46,11.92 v57.84,9.54
  pour Top (isolate 0.61): 15.55,13.7 15.49,-0.75 74.88,-0.86 68.8,13.67
VCAP_1
  Top 0.254: U$1.VCAP_1 44.25,15.4 44.65,15 C_VCAP1.2
VCAP_2
  Top 0.254: U$1.VCAP_2 47.68,25.25 47.92,25.01 C_VCAP2.1
VMTR
  Top 0.305: R_VMTR_1.2 14,13.55 R_VMTR_2.1 16.02,15.53 31.38,15.53 32.44,14.47 41.72,14.47 42.25,15 U$1.PB1

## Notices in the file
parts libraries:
SparkFun-Capacitors: Licensing: Creative Commons ShareAlike 4.0 International - https://creativecommons.org/licenses/by-sa/4.0
